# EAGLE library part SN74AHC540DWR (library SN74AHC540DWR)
Octal Buffers/Drivers With 3-State Outputs Source: Datasheet
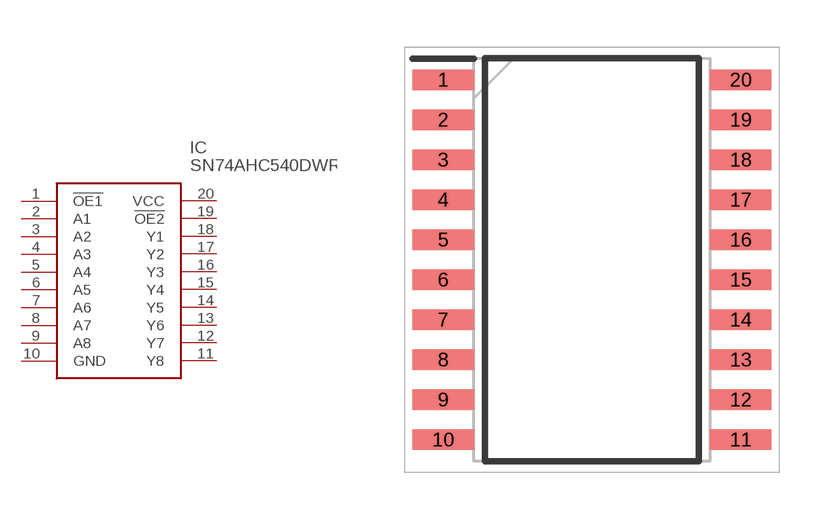
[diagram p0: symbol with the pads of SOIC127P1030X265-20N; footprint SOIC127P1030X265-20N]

Designator prefix IC

## SN74AHC540DWR (Description: Octal Buffers/Drivers With 3-State Outputs; Height: 2.65mm; Manufacturer_Name: Texas Instruments; Manufacturer_Part_Number: SN74AHC540DWR; Mouser_Part_Number: 595-SN74AHC540DWR; Mouser_Price-Stock: https://www.mouser.com/Search/Refine.aspx?Keyword=595-SN74AHC540DWR)  [SOIC127P1030X265-20N]
1  !OE1
2  A1
3  A2
4  A3
5  A4
6  A5
7  A6
8  A7
9  A8
10  GND
11  Y8
12  Y7
13  Y6
14  Y5
15  Y4
16  Y3
17  Y2
18  Y1
19  !OE2
20  VCC

## Footprint SOIC127P1030X265-20N (pad centres in mm)
DW0020A
smd 1.95 x 0.65: 1 -4.725,5.715; 2 -4.725,4.445; 3 -4.725,3.175; 4 -4.725,1.905; 5 -4.725,0.635; 6 -4.725,-0.635; 7 -4.725,-1.905; 8 -4.725,-3.175; 9 -4.725,-4.445; 10 -4.725,-5.715; 11 4.725,-5.715; 12 4.725,-4.445; 13 4.725,-3.175; 14 4.725,-1.905; 15 4.725,-0.635; 16 4.725,0.635; 17 4.725,1.905; 18 4.725,3.175; 19 4.725,4.445; 20 4.725,5.715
